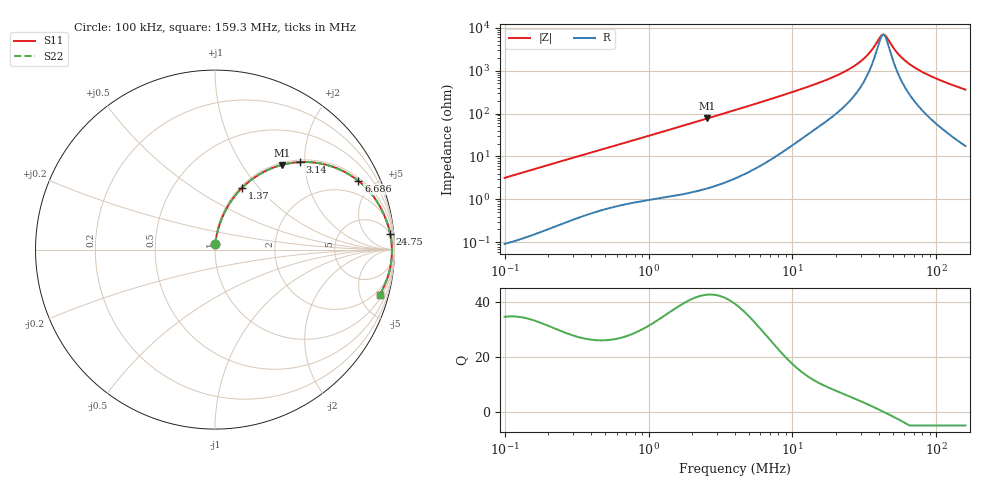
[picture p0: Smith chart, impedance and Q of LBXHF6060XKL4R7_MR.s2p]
! LBXHF6060XKL4R7_MR  S-PARAMETER MODEL  ( General Type )
! Model Generated by TAIYO YUDEN Corporation (http://www.ty-top.com)
! Version 1.0
! TAIYO YUDEN Control No. 220210
! Copyright(c) 2022 TAIYO YUDEN CO.,LTD. All Rights Reserved.
! Product Description (link to TY-COMPAS)
! https://ds.yuden.co.jp/TYCOMPAS/or/detail?pn=LBXHF6060XKL4R7MMR&u=M
! Products Name : Inductors
! Characteristics :
!  Inductance : 4.7 uH , SRF(min) : 30 MHz , DC Resistance(max) : 0.036 Ohm
!  Rated Current : Saturation :3300 mA , Temp Rise : 3800 mA
!  Case Size : 6.0 x 6.0 / 0.236 x 0.236 [mm/inch] , Thickness : 3 / 0.118 [mm/inch]
!  (Conditions: Temperature = 25 degC , DC Bias Current/Voltage = 0A / 0V)
! External Node Assignments :
!  1  o---GGG---o  2
! GND o---------o GND
! Frequency Range : 0.1MHz  -  159.254811MHz  [ 402 STEP ]
# MHz S RI R 50
! Freq[MHz].  S11 Real  S11 Imag  S21 Real  S21 Imag  S12 Real  S12 Imag  S22 Real  S22 Imag
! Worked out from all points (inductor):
!   401 points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, 100 kHz to 159.3 MHz, reference 50 ohm
!   read as one part in series: L = 5.04 uH near 103.8 kHz
!   highest Q = 42.5 at 2.564 MHz (marker M1), where L = 4.77 uH
!   self-resonance near 42.24 MHz
!   S11 on the Smith chart (normalised r, x): 100 kHz: 1.00, +0.06; 1.37 MHz: 1.02, +0.82; 3.14 MHz: 1.04, +1.88; 6.686 MHz: 1.15, +4.10; 24.75 MHz: 5, +21; 159.3 MHz: 1.35, -7.19
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0.1  0.00193 0.0317  0.9981 -0.0317  0.9981 -0.0317  0.00193 0.0317
0.343835  0.0151 0.1049  0.9849 -0.1049  0.9849 -0.1049  0.0151 0.1049
0.705593  0.0508 0.202  0.9492 -0.202  0.9492 -0.202  0.0508 0.202
1.182227  0.1194 0.3097  0.8806 -0.3097  0.8806 -0.3097  0.1194 0.3097
1.37007  0.1515 0.3449  0.8485 -0.3449  0.8485 -0.3449  0.1515 0.3449
2.564016  0.3739 0.4722  0.6261 -0.4722  0.6261 -0.4722  0.3739 0.4722
3.140352  0.4709 0.4874  0.5291 -0.4874  0.5291 -0.4874  0.4709 0.4874
4.064915  0.5973 0.4777  0.4027 -0.4777  0.4027 -0.4777  0.5973 0.4777
6.686406  0.799 0.3828  0.201 -0.3828  0.201 -0.3828  0.799 0.3828
13.72135  0.9384 0.2017  0.0616 -0.2017  0.0616 -0.2017  0.9384 0.2017
19.12014  0.9641 0.1341  0.0359 -0.1341  0.0359 -0.1341  0.9641 0.1341
24.74937  0.9761 0.0879  0.0239 -0.0879  0.0239 -0.0879  0.9761 0.0879
28.68178  0.9805 0.0633  0.0195 -0.0633  0.0195 -0.0633  0.9805 0.0633
32.63192  0.9832 0.0425  0.0168 -0.0425  0.0168 -0.0425  0.9832 0.0425
35.78235  0.9845 0.028  0.0155 -0.028  0.0155 -0.028  0.9845 0.028
41.46777  0.9857 0.00497  0.0143 -0.00497  0.0143 -0.00497  0.9857 0.00497
43.82545  0.9858 -0.00364  0.0142 0.00364  0.0142 0.00364  0.9858 -0.00364
47.17884  0.9857 -0.0151  0.0143 0.0151  0.0143 0.0151  0.9857 -0.0151
55.6922  0.9844 -0.0414  0.0156 0.0414  0.0156 0.0414  0.9844 -0.0414
70.77215  0.9797 -0.0813  0.0203 0.0813  0.0203 0.0813  0.9797 -0.0813
100.4527  0.9643 -0.1467  0.0357 0.1467  0.0357 0.1467  0.9643 -0.1467
159.2548  0.918 -0.2512  0.082 0.2512  0.082 0.2512  0.918 -0.2512
